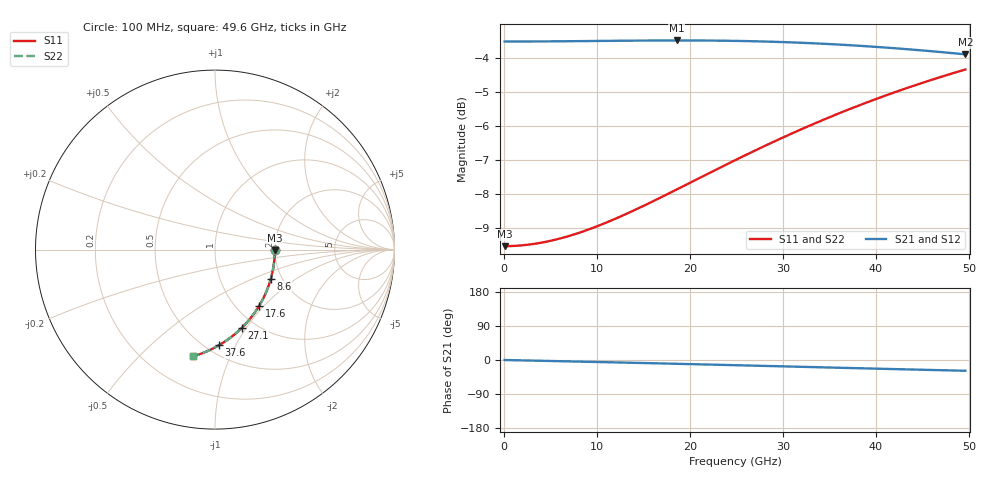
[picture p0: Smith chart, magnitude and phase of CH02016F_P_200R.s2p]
# GHz S RI R 200
! S-Parameters data
! Freq  reS11  imS11  reS21  imS21  reS12  imS12  reS22  imS22
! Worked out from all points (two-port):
!   100 points, 100 MHz to 49.6 GHz, reference 200 ohm
!   highest |S21| = -3.49 dB at 18.6 GHz (marker M1); lowest = -3.9 dB at 49.6 GHz (marker M2)
!   |S21| within 3 dB of the highest: start of sweep to end of sweep
!   lowest |S11| = -9.5 dB at 100 MHz (marker M3), VSWR 2.00, Z = 400 - j1.72 ohm
!   |S11| at or under -10 dB: nowhere
!   |S22| runs from -9.5 to -4.3 dB; largest |S21 - S12| = 0
!   S11 on the Smith chart (normalised r, x): 100 MHz: 2.00, -0.01; 8.6 GHz: 1.75, -0.65; 17.6 GHz: 1.27, -0.94; 27.1 GHz: 0.86, -0.95; 37.6 GHz: 0.58, -0.86; 49.6 GHz: 0.39, -0.74
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0.1  0.3333 -0.00191  0.6667 -0.0006  0.6667 -0.0006  0.3333 -0.00191
2.1  0.332 -0.0401  0.6666 -0.0126  0.6666 -0.0126  0.332 -0.0401
4.1  0.3282 -0.0781  0.6665 -0.0247  0.6665 -0.0247  0.3282 -0.0781
6.1  0.3221 -0.1156  0.6662 -0.0369  0.6662 -0.0369  0.3221 -0.1156
8.6  0.3113 -0.1614  0.6656 -0.0523  0.6656 -0.0523  0.3113 -0.1614
10.6  0.3003 -0.197  0.6649 -0.0648  0.6649 -0.0648  0.3003 -0.197
12.6  0.2872 -0.2315  0.6639 -0.0774  0.6639 -0.0774  0.2872 -0.2315
14.6  0.2723 -0.2647  0.6626 -0.0903  0.6626 -0.0903  0.2723 -0.2647
16.6  0.2557 -0.2964  0.6609 -0.1034  0.6609 -0.1034  0.2557 -0.2964
17.6  0.2468 -0.3118  0.6599 -0.1099  0.6599 -0.1099  0.2468 -0.3118
18.6  0.2376 -0.3267  0.6588 -0.1165  0.6588 -0.1165  0.2376 -0.3267
22.1  0.2028 -0.3758  0.654 -0.1398  0.654 -0.1398  0.2028 -0.3758
25.1  0.1705 -0.4139  0.6486 -0.1599  0.6486 -0.1599  0.1705 -0.4139
27.1  0.1479 -0.4371  0.6443 -0.1732  0.6443 -0.1732  0.1479 -0.4371
30.1  0.1129 -0.4689  0.6367 -0.1929  0.6367 -0.1929  0.1129 -0.4689
33.1  0.0771 -0.497  0.6279 -0.2122  0.6279 -0.2122  0.0771 -0.497
35.1  0.0528 -0.5138  0.6214 -0.2247  0.6214 -0.2247  0.0528 -0.5138
37.6  0.0224 -0.5327  0.6126 -0.2399  0.6126 -0.2399  0.0224 -0.5327
39.6  -0.00195 -0.5461  0.605 -0.2516  0.605 -0.2516  -0.00195 -0.5461
41.6  -0.0262 -0.5582  0.597 -0.2629  0.597 -0.2629  -0.0262 -0.5582
45.6  -0.0742 -0.5785  0.5798 -0.2842  0.5798 -0.2842  -0.0742 -0.5785
49.6  -0.121 -0.5942  0.5615 -0.3036  0.5615 -0.3036  -0.121 -0.5942
